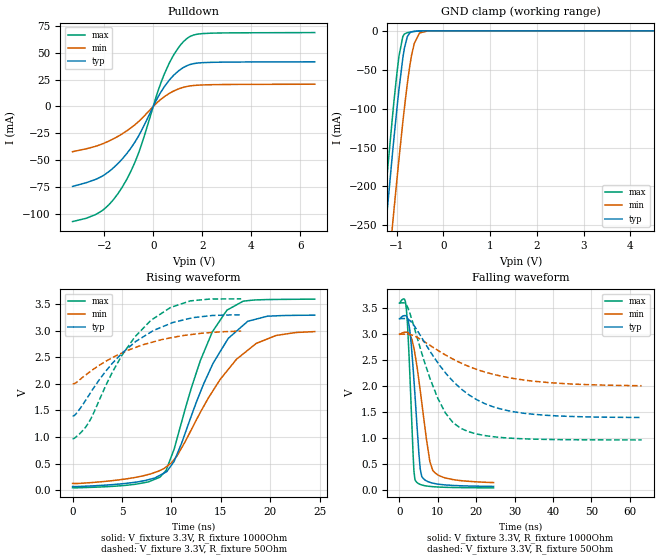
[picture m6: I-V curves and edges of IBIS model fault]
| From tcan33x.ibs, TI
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|   fault Model
[Model]   fault
Model_type   Open_drain
Polarity   Non-Inverting
Vmeas = 1.65
Vref = 3.3
Cref = 2pF
Rref = 1000
|   typ   min   max
|   (nom PVT)   (fast PVT)   (slow PVT)
C_comp   1.225e-12   1.198e-12   1.298e-12
| Where nom  PVT is Nominal Process, 3.3V, 27C
|   Fast PVT is Strong Process,  3.6V, -40C
|   Slow PVT is Weak Process,   3V, 150C
[Voltage Range]   3.3   3   3.6
|Junction Temperature
[Temperature Range]   27   150   -40
[Pullup Reference]   3.3   3   3.6
[Pulldown Reference]   0   0   0
[Power Clamp Reference]   3.3   3   3.6
[GND Clamp Reference]   0   0   0
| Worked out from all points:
|   slope of the pulldown table from 0 to 0.495 V, typ, clamps not added: 25.2 ohm
|   GND clamp passes 1 mA (typ) near -0.66 V on its own axis
|   falling waveform, V_fixture 3.3V, R_fixture 1000Ohm: 20-80 % time 1.82ns typ, 3.11ns min, 1.22ns max; typ from 3.3 V to 0.076 V
|   rising waveform, V_fixture 3.3V, R_fixture 1000Ohm: 20-80 % time 4.41ns typ, 5.63ns min, 3.69ns max; typ from 0.069 V to 3.29 V
|   falling waveform, V_fixture 3.3V, R_fixture 50Ohm: 20-80 % time 13.4ns typ, 18ns min, 7.83ns max; typ from 3.3 V to 1.4 V
|   rising waveform, V_fixture 3.3V, R_fixture 50Ohm: 20-80 % time 5.81ns typ, 6.72ns min, 5.05ns max; typ from 1.4 V to 3.3 V
[Pulldown]
|   Voltage   I(typ)   I(min)   I(max)
-3.3V     -74.46mA   -42.16mA   -107.2mA
-2.123V   -65.37mA   -35.27mA   -97.48mA
-1.674V   -58.05mA   -30.71mA   -87.97mA
-1.28V    -49.21mA   -25.67mA   -75.54mA
-927mV    -39.16mA   -20.2mA    -60.88mA
-615mV    -28.08mA   -14.39mA   -44.22mA
147mV     6.789mA    3.357mA    11.17mA
462mV     18.66mA    9.239mA    30.71mA
858mV     29.54mA    14.58mA    48.83mA
1.369V    37.83mA    18.51mA    63.07mA
2.042V    40.75mA    20mA       67.82mA
6.6V      41.5mA     20.66mA    68.72mA
[GND Clamp]
|   Voltage   I(typ)   I(min)   I(max)
-3.3V     -1.72A     -1.582A    -1.813A
-1.399V   -362.1mA   -453mA     -316.5mA
-1.287V   -286mA     -378.4mA   -239.3mA
-1.075V   -148.3mA   -241.1mA   -100.9mA
-949.2mV  -74.28mA   -163.8mA   -31.97mA
-867.9mV  -34.69mA   -117.1mA   -7.272mA
-772.2mV  -7.558mA   -67.8mA    -2.328mA
-676.5mV  -1.227mA   -29.86mA   -1.233mA
-620.4mV  -631.5uA   -15.73mA   -754uA
-510mV    -168.9uA   -2.707mA   -173.7uA
-330mV    -5.144uA   -45.34uA   -2.545uA
6.6V      0A         0A         0A
[POWER Clamp]
|   Voltage   I(typ)   I(min)   I(max)
-3.3V     0A         0A         0A
0V        0A         0A         0A
6.6V      0A         0A         0A
[Ramp]
R_load = 1000
|   typ   min   max
dV/dt_r   1.93835/4.42859e-09   1.7236/5.67631e-09   2.13236/3.69619e-09
dV/dt_f   1.93833/1.82324e-09   1.7236/3.13966e-09   2.13228/1.22052e-09
[Falling Waveform]
V_fixture = 3.3V
V_fixture_min = 3V
V_fixture_max = 3.6V
R_fixture = 1000Ohm
|   Time   V(typ)   V(min)   V(max)
0s        3.3V       3V         3.6V
1.339ns   3.359V     3.04V      3.674V
1.839ns   3.346V     3.04V      3.465V
2.663ns   3.101V     2.998V     2.313V
3.567ns   2.344V     2.801V     678.1mV
4.037ns   1.84V      2.625V     206.9mV
5.429ns   403.4mV    1.912V     113.5mV
7.92ns    154.6mV    553.9mV    75.72mV
8.672ns   138.8mV    382.8mV    70.77mV
24.5ns    75.76mV    149.5mV    48.04mV
[Rising Waveform]
V_fixture = 3.3V
V_fixture_min = 3V
V_fixture_max = 3.6V
R_fixture = 1000Ohm
|   Time   V(typ)   V(min)   V(max)
0s        69.42mV    127.3mV    46.11mV
6.483ns   153.8mV    245.5mV    114.6mV
8.839ns   280.7mV    371.5mV    244.3mV
9.465ns   342.7mV    438.2mV    372.2mV
10.27ns   539.8mV    575.9mV    769.2mV
12.95ns   1.854V     1.47V      2.446V
14.13ns   2.354V     1.851V     2.976V
15.62ns   2.817V     2.242V     3.388V
18.58ns   3.219V     2.761V     3.58V
24.5ns    3.293V     2.984V     3.594V
[Falling Waveform]
V_fixture = 3.3V
V_fixture_min = 3V
V_fixture_max = 3.6V
R_fixture = 50Ohm
|   Time   V(typ)   V(min)   V(max)
0s        3.3V       3V         3.6V
1.558ns   3.303V     3.002V     3.593V
2.218ns   3.292V     3V         3.507V
6.296ns   2.874V     2.867V     2.519V
9.929ns   2.458V     2.694V     1.78V
11.93ns   2.264V     2.605V     1.492V
15.93ns   1.96V      2.451V     1.194V
22.19ns   1.668V     2.277V     1.054V
30.19ns   1.505V     2.145V     997.7mV
63.06ns   1.401V     2.011V     969.1mV
[Rising Waveform]
V_fixture = 3.3V
V_fixture_min = 3V
V_fixture_max = 3.6V
R_fixture = 50Ohm
|   Time   V(typ)   V(min)   V(max)
0s        1.397V     2.002V     968.6mV
476ps     1.466V     2.041V     1.022V
1.558ns   1.759V     2.201V     1.249V
3.984ns   2.379V     2.489V     2.205V
4.99ns    2.575V     2.581V     2.537V
6.296ns   2.782V     2.68V      2.882V
7.929ns   2.975V     2.777V     3.197V
9.929ns   3.138V     2.866V     3.439V
11.93ns   3.235V     2.927V     3.562V
17.06ns   3.298V     2.993V     3.599V
